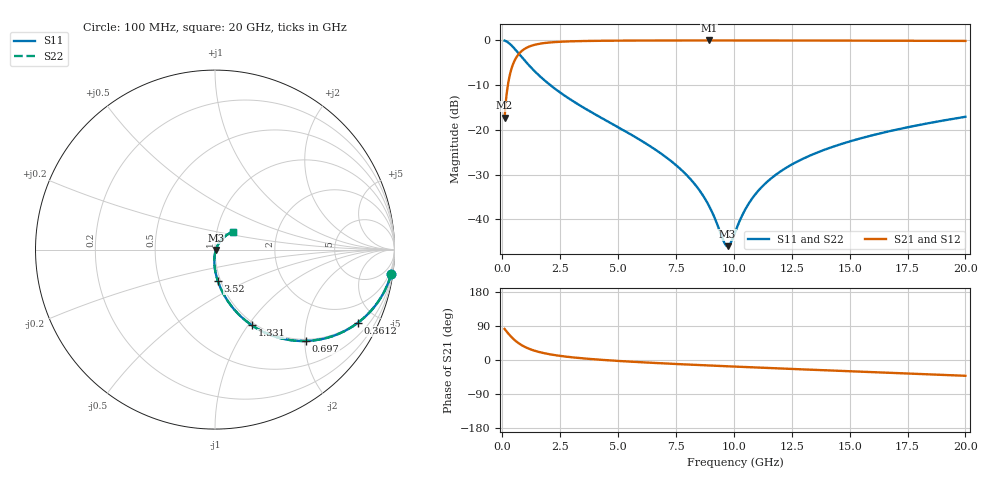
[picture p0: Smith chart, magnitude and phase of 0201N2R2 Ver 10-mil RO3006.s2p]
# GHz S MA R 50
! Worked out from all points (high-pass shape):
!   1601 points, 100 MHz to 20 GHz, reference 50 ohm
!   highest |S21| = -0.05 dB at 8.931 GHz (marker M1); lowest = -17.3 dB at 100 MHz (marker M2)
!   |S21| within 3 dB of the highest: 715.7 MHz to end of sweep
!   lowest |S11| = -46.0 dB at 9.727 GHz (marker M3), VSWR 1.01, Z = 50.5 - j0.151 ohm
!   |S11| at or under -10 dB: 2.07 GHz to end of sweep
!   |S22| runs from -46.0 to -0.1 dB; largest |S21 - S12| = 0
!   S11 on the Smith chart (normalised r, x): 100 MHz: 1, -14; 361.2 MHz: 0.96, -3.91; 697 MHz: 0.96, -2.02; 1.331 GHz: 0.96, -1.04; 3.52 GHz: 0.97, -0.35; 20 GHz: 1.19, +0.24
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0.1  0.9905 -8.0  0.137 81.9  0.137 81.9  0.9905 -8.0
0.2616875  0.94 -20.3  0.3403 69.6  0.3403 69.6  0.94 -20.3
0.3611875  0.894 -27.2  0.447 62.8  0.447 62.8  0.894 -27.2
0.697  0.7175 -45.2  0.6948 44.7  0.6948 44.7  0.7175 -45.2
0.9955  0.5829 -55.8  0.8103 33.9  0.8103 33.9  0.5829 -55.8
1.331312  0.4698 -64.0  0.8803 25.7  0.8803 25.7  0.4698 -64.0
2.114875  0.3097 -75.0  0.9478 14.4  0.9478 14.4  0.3097 -75.0
3.420812  0.1828 -84.2  0.9796 4.7  0.9796 4.7  0.1828 -84.2
3.520313  0.1764 -84.7  0.9807 4.1  0.9807 4.1  0.1764 -84.7
6.741625  0.05705 -93.9  0.9938 -8.3  0.9938 -8.3  0.05705 -93.9
8.047562  0.02966 -93.0  0.9947 -12.1  0.9947 -12.1  0.02966 -93.0
8.930625  0.01414 -84.3  0.9948 -14.5  0.9948 -14.5  0.01414 -84.3
9.5525  0.005764 -46.0  0.9948 -16.1  0.9948 -16.1  0.005764 -46.0
9.726625  0.005033 -17.3  0.9947 -16.6  0.9947 -16.6  0.005033 -17.3
9.863437  0.005483 5.7  0.9947 -17.0  0.9947 -17.0  0.005483 5.7
10.05  0.007173 27.3  0.9946 -17.4  0.9946 -17.4  0.007173 27.3
10.58481  0.01422 49.8  0.9944 -18.8  0.9944 -18.8  0.01422 49.8
11.244  0.02357 56.5  0.9941 -20.5  0.9941 -20.5  0.02357 56.5
12.16437  0.03641 58.6  0.9936 -22.8  0.9936 -22.8  0.03641 58.6
13.37081  0.05274 58.1  0.9926 -25.7  0.9926 -25.7  0.05274 58.1
16.69162  0.09621 52.5  0.9887 -33.7  0.9887 -33.7  0.09621 52.5
20  0.1399 45.5  0.9828 -41.7  0.9828 -41.7  0.1399 45.5
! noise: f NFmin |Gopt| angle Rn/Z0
0.1  0.0009592  0.9559  0.6047  0.0049
2.301  0.005358  0.8259  4.263  0.00646
4.515  0.008286  0.7843  7.957  0.007855
6.729  0.01081  0.7577  11.65  0.008938
8.943  0.01312  0.7383  15.31  0.009856
11.14  0.01527  0.7233  18.92  0.01067
13.36  0.01735  0.7113  22.52  0.01141
15.57  0.01937  0.7017  26.07  0.01209
17.79  0.02135  0.6938  29.58  0.01274
20  0.02331  0.6876  33.05  0.01336
